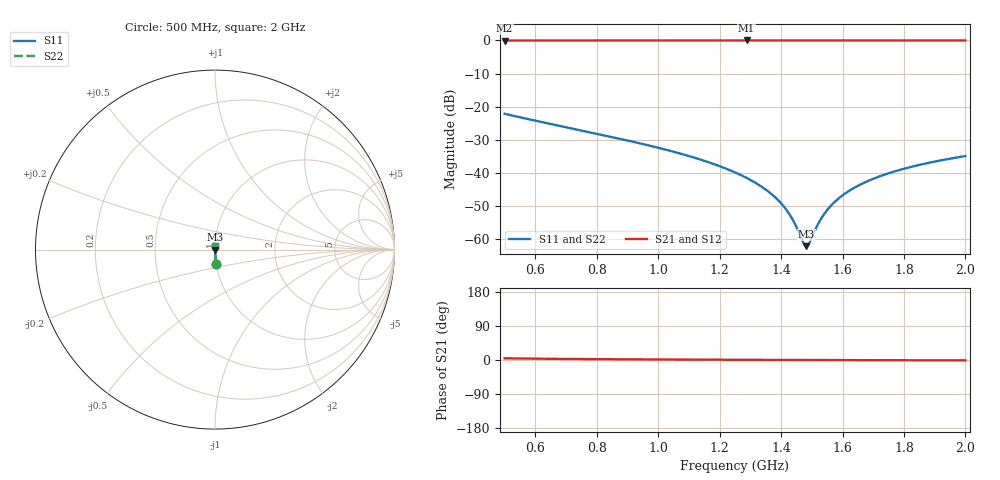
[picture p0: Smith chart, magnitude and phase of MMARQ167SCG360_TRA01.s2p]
! MMARQ167SCG360_TRA01  S-PARAMETER MODEL  ( General Type )
! Model Generated by TAIYO YUDEN Corporation (http://www.ty-top.com)
! Version 1.0
! TAIYO YUDEN Control No. 160201
! Copyright(c) 2016 TAIYO YUDEN CO.,LTD. All Rights Reserved.
! Product Description (link to TY-COMPAS)
! https://ds.yuden.co.jp/TYCOMPAS/or/detail?pn=MMARQ167SCG360JTRA01&u=M
! Products Name : Multilayer Ceramic Capacitors
! Characteristics :
!  Capacitance : 36 pF , Rated Voltage : 250V , TCC : CG / C0G
!  Case Size : 1.6 x 0.8 / 0.063 x 0.031 [mm/inch] , Thickness : 0.7 / 0.028 [mm/inch]
!  (Conditions: Temperature = 25 degC , DC Bias Current/Voltage = 0A / 0V)
! External Node Assignments :
!  1  o---| |---o  2
! GND o---------o GND
! Frequency Range : 500MHz  -  2000MHz  [ 401 STEP ]
# MHz S RI R 50
! Freq[MHz].  S11 Real  S11 Imag  S21 Real  S21 Imag  S12 Real  S12 Imag  S22 Real  S22 Imag
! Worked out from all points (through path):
!   401 points, 500 MHz to 2 GHz, reference 50 ohm
!   highest |S21| = -0.01 dB at 1.288 GHz (marker M1); lowest = 0.0 dB at 500 MHz (marker M2)
!   lowest |S11| = -62.1 dB at 1.482 GHz (marker M3), VSWR 1.00, Z = 50.1 - j0.000584 ohm
!   |S11| at or under -10 dB: start of sweep to end of sweep
!   |S22| runs from -62.1 to -22.1 dB; largest |S21 - S12| = 0
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500  0.00643 -0.0779  0.9936 0.0779  0.9936 0.0779  0.00643 -0.0779
751.25  0.00236 -0.0435  0.9976 0.0435  0.9976 0.0435  0.00236 -0.0435
1002.5  0.00116 -0.0238  0.9988 0.0238  0.9988 0.0238  0.00116 -0.0238
1141.25  0.0009 -0.0157  0.9991 0.0157  0.9991 0.0157  0.0009 -0.0157
1250  0.000803 -0.0102  0.9992 0.0102  0.9992 0.0102  0.000803 -0.0102
1287.5  0.000784 -0.00838  0.9992 0.00838  0.9992 0.00838  0.000784 -0.00838
1351.25  0.000768 -0.0055  0.9992 0.0055  0.9992 0.0055  0.000768 -0.0055
1400  0.000767 -0.00339  0.9992 0.00339  0.9992 0.00339  0.000767 -0.00339
1430  0.000771 -0.00214  0.9992 0.00214  0.9992 0.00214  0.000771 -0.00214
1445  0.000774 -0.00152  0.9992 0.00152  0.9992 0.00152  0.000774 -0.00152
1471.25  0.00078 -0.000456  0.9992 0.000456  0.9992 0.000456  0.00078 -0.000456
1482.5  0.000784 -5.84e-06  0.9992 5.84e-06  0.9992 5.84e-06  0.000784 -5.84e-06
1490  0.000786 0.000292  0.9992 -0.000292  0.9992 -0.000292  0.000786 0.000292
1501.25  0.00079 0.000737  0.9992 -0.000737  0.9992 -0.000737  0.00079 0.000737
1520  0.000798 0.00147  0.9992 -0.00147  0.9992 -0.00147  0.000798 0.00147
1538.75  0.000806 0.0022  0.9992 -0.0022  0.9992 -0.0022  0.000806 0.0022
1561.25  0.000818 0.00305  0.9992 -0.00305  0.9992 -0.00305  0.000818 0.00305
1587.5  0.000833 0.00404  0.9992 -0.00404  0.9992 -0.00404  0.000833 0.00404
1658.75  0.000881 0.00664  0.9991 -0.00664  0.9991 -0.00664  0.000881 0.00664
1752.5  0.00096 0.00992  0.999 -0.00992  0.999 -0.00992  0.00096 0.00992
1865  0.00108 0.0137  0.9989 -0.0137  0.9989 -0.0137  0.00108 0.0137
2000  0.00124 0.0179  0.9988 -0.0179  0.9988 -0.0179  0.00124 0.0179
